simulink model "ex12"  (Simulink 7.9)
settings: Solver=ode45  StartTime=0.0  StopTime=simulation_time  RelTol=1e-3
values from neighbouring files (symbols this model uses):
  a = 1    [ex12init.m]    (also in ex13init.m)
  am = 2    [ex12init.m]    (also in ex13init.m)
  b = 0.5    [ex12init.m]    (also in ex13init.m)
  bm = 2    [ex12init.m]    (also in ex13init.m)
  gamma = 1    [ex12init.m]    (also in ex11init.m)
libraries: simulink x1

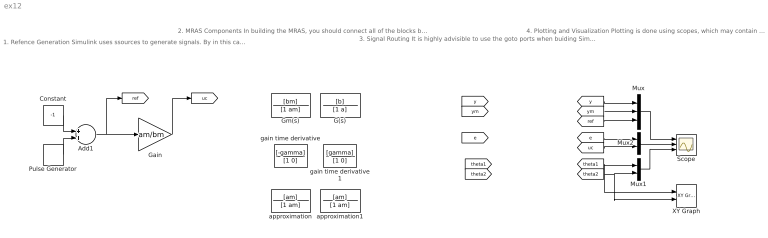
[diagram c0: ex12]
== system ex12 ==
  note: 1. Refence Generation Simulink uses ssources to generate signals. By in this case using a pulse generator which is shifted. In order to yield unit static gain from reference to output, the reference is scaled by a parameter 1/k0 to generate the controlled input u_c
  note: 2. MRAS Components In building the MRAS, you should connect all of the blocks below as shown in Figure 1. These blocks are all instances of continuous time transfer function blocks, locatred in the library browser.
  note: 3. Signal Routing It is highly advisible to use the goto ports when buiding Simulink models, especially with more complex controllers. Connect these goto ports to the corresponding signals in your system
  note: 4. Plotting and Visualization Plotting is done using scopes, which may contain several axis. To combine signals in the same view, the variants of the mux operator can be used. Double click scope to see the signals.
  Add1 : Sum
  Constant : Constant  Value=-1  SampleTime=0.1
  G(s) : TransferFcn  Numerator=[b]  Denominator=[1 a]
  Gain : Gain  Gain=am/bm
  Gm(s) : TransferFcn  Numerator=[bm]  Denominator=[1 am]
  Mux : Mux  Inputs=3
  Mux1 : Mux  Inputs=2
  Mux2 : Mux  Inputs=2
  Pulse Generator : DiscretePulseGenerator  PulseType=Time based  Amplitude=2  Period=10  PulseWidth=50
  Scope : Scope  NumInputPorts=3
  XY Graph : simulink/Sinks/XY Graph  xmin=-8  xmax=8  ymin=-8  ymax=8  st=-1
  approximation : TransferFcn  Numerator=[am]  Denominator=[1 am]
  approximation1 : TransferFcn  Numerator=[am]  Denominator=[1 am]
  gain time derivative : TransferFcn  Numerator=[-gamma]  Denominator=[1 0]
  gain time derivative1 : TransferFcn  Numerator=[gamma]  Denominator=[1 0]
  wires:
  [y] -> Mux/1
  Mux/1 -> Scope/1
  [ym] -> Mux/2
  [ref] -> Mux/3
  Constant/1 -> Add1/1
  Pulse Generator/1 -> Add1/2
  Add1/1 -> Gain/1, [ref]
  [theta2] -> Mux1/2, XY Graph/2
  [theta1] -> Mux1/1, XY Graph/1
  Mux1/1 -> Scope/3
  [e] -> Mux2/1
  [uc] -> Mux2/2
  Mux2/1 -> Scope/2
  Gain/1 -> [uc]
